FUNCTION_BLOCK Example17_cam //4x3 flyways 2 xbot sample cam set as cam 128 (position interval = 1 mm) - cam mode, cam mode advanced
VAR_INPUT
	Execute : BOOL;
END_VAR
VAR_OUTPUT
	Done : BOOL;
END_VAR
VAR_IN_OUT
	PM_Controller : PMControllerType;	// the planar motor controller to use
END_VAR
VAR
	xbotID_array78 : ARRAY[0..77] OF USINT;
	PosX_array78 : ARRAY[0..77] OF REAL;
	PosY_array78 : ARRAY[0..77] OF REAL;
	PMC_AutoDrivingMotion1 : PMC_AutoDrivingMotion;
	slave_axis_array7 : ARRAY[0..6] OF USINT;
	cam_ID_array7 : ARRAY[0..6] OF USINT;
	master_xbot_ID_array7 : ARRAY[0..6] OF USINT;
	master_axis_array7 : ARRAY[0..6] OF USINT;
	PMC_CamModeCtrl1 : PMC_CamModeCtrl;
	PMC_XYMotion1 : PMC_XYMotion;
	PMC_XYMotion2 : PMC_XYMotion;
	PMC_CamModeCtrl2 : PMC_CamModeCtrl;
	PMC_AutoDrivingMotion2 : PMC_AutoDrivingMotion;
	SlaveAID_array4 : ARRAY[0..3] OF USINT;
	camID_array4 : ARRAY[0..3] OF USINT;
	MasterXID_array4 : ARRAY[0..3] OF USINT;
	MasterAID_array4 : ARRAY[0..3] OF USINT;
	MasterAOffset_array4 : ARRAY[0..3] OF REAL;
	SlaveAOffset_array4 : ARRAY[0..3] OF REAL;
	MasterAScaling_array4 : ARRAY[0..3] OF REAL;
	SlaveAScaling_array4 : ARRAY[0..3] OF REAL;
	CamMode_array4 : ARRAY[0..3] OF USINT;
	MasterOffsetMode_array4 : ARRAY[0..3] OF USINT;
	PMC_CamModeCtrlAdvanced1 : PMC_CamModeCtrlAdvanced;
	PMC_XYMotion3 : PMC_XYMotion;
	PMC_XYMotion4 : PMC_XYMotion;
	PMC_CamModeCtrlAdvanced2 : PMC_CamModeCtrlAdvanced;
END_VAR

//4x3 flyways 2 xbot sample cam set as cam 128 (position interval = 1 mm) - cam mode, cam mode advanced

//move async move to 60,60 and 60,180
xbotID_array78[0] := 1;xbotID_array78[1] := 2;
PosX_array78[0] := 0.06;PosX_array78[1] := 0.06;
PosY_array78[0] := 0.06;PosY_array78[1] := 0.18;
PMC_AutoDrivingMotion1(Execute := Execute,nXbots := 2,XbotID := xbotID_array78,RoutingType := 0,ZoneID := 0,PosX := PosX_array78,PosY := PosY_array78,PM_Controller := PM_Controller);

//setup cam with xbot 2 y as slave to xbot 1 x
slave_axis_array7[0] := 2;
cam_ID_array7[0] := 128;
master_xbot_ID_array7[0] := 1;
master_axis_array7[0] := 1;
PMC_CamModeCtrl1(Execute := PMC_AutoDrivingMotion1.Done,cmdLB := 2,Level := 1,SlaveXID := 2,nAxis := 1,SlaveAID := slave_axis_array7,camID := cam_ID_array7,MasterXID := master_xbot_ID_array7,MasterAID := master_axis_array7,PM_Controller := PM_Controller);

//move xbot 1 to (400,60)
PMC_XYMotion1(Execute := PMC_CamModeCtrl1.Done,cmdLB := 3,XbotID := 1,Mode := 0,Type_ := 0,PosX := 0.4,PosY := 0.06,EndVel := 0,MaxVel := 0.25,MaxAcc := 10,PM_Controller := PM_Controller);

//move xbot 1 to (60,60)
PMC_XYMotion2(Execute := PMC_XYMotion1.Done,cmdLB := 4,XbotID := 1,Mode := 0,Type_ := 0,PosX := 0.06,PosY := 0.06,EndVel := 0,MaxVel := 0.25,MaxAcc := 10,PM_Controller := PM_Controller);

//disable cam on xbot 2 
PMC_CamModeCtrl2(Execute := PMC_XYMotion2.Done,cmdLB := 5,Level := 0,SlaveXID := 2,nAxis := 1,SlaveAID := slave_axis_array7,camID := cam_ID_array7,MasterXID := master_xbot_ID_array7,MasterAID := master_axis_array7,PM_Controller := PM_Controller);

//move to new start position (60,60) and (480,420)
xbotID_array78[0] := 1;xbotID_array78[1] := 2;
PosX_array78[0] := 0.06;PosX_array78[1] := 0.48;
PosY_array78[0] := 0.06;PosY_array78[1] := 0.42;
PMC_AutoDrivingMotion2(Execute := PMC_CamModeCtrl2.Done,nXbots := 2,RoutingType := 0,ZoneID := 0,XbotID := xbotID_array78,PosX := PosX_array78,PosY := PosY_array78,PM_Controller := PM_Controller);

//setup advanced cam
SlaveAID_array4[0] := 1; SlaveAID_array4[1] := 2;
camID_array4[0] := 128; camID_array4[1] := 128;
MasterXID_array4[0] := 1; MasterXID_array4[1] := 1;
MasterAID_array4[0] := 1;MasterAID_array4[1] := 1;
MasterAOffset_array4[0] := 0; MasterAOffset_array4[1] := 0;
SlaveAOffset_array4[0] := 0; SlaveAOffset_array4[1] := 0;
MasterAScaling_array4[0] := 1; MasterAScaling_array4[1] := 2;
SlaveAScaling_array4[0] := 2; SlaveAScaling_array4[1] := 1;
CamMode_array4[0] := 1; CamMode_array4[1] := 1;
MasterOffsetMode_array4[0] := 1; MasterOffsetMode_array4[1] := 1;
PMC_CamModeCtrlAdvanced1(Execute := PMC_AutoDrivingMotion2.Done,cmdLB := 6,Level := 1,SlaveXID := 2,nAxis := 2,SlaveAID := SlaveAID_array4,camID := camID_array4,
						MasterXID := MasterXID_array4,MasterAID := MasterAID_array4,MasterAOffset := MasterAOffset_array4,SlaveAOffset := SlaveAOffset_array4,
						MasterAScaling := MasterAScaling_array4,SlaveAScaling := SlaveAScaling_array4,CamMode := CamMode_array4,MasterOffsetMode := MasterOffsetMode_array4,PM_Controller := PM_Controller);
						
//move xbot 1 to (400,60)
PMC_XYMotion3(Execute := PMC_CamModeCtrlAdvanced1.Done,cmdLB := 7,XbotID := 1,Mode := 0,Type_ := 0,PosX := 0.9,PosY := 0.06,EndVel := 0,MaxVel := 0.25,MaxAcc := 10,PM_Controller := PM_Controller);

//move xbot 1 to (60,60)
PMC_XYMotion4(Execute := PMC_XYMotion3.Done,cmdLB := 8,XbotID := 1,Mode := 0,Type_ := 0,PosX := 0.06,PosY := 0.06,EndVel := 0,MaxVel := 0.25,MaxAcc := 10,PM_Controller := PM_Controller);

//disable advanced cam
PMC_CamModeCtrlAdvanced2(Execute := PMC_XYMotion4.Done,cmdLB := 9,Level := 0,SlaveXID := 2,nAxis := 2,SlaveAID := SlaveAID_array4,camID := camID_array4,
						MasterXID := MasterXID_array4,MasterAID := MasterAID_array4,MasterAOffset := MasterAOffset_array4,SlaveAOffset := SlaveAOffset_array4,
						MasterAScaling := MasterAScaling_array4,SlaveAScaling := SlaveAScaling_array4,CamMode := CamMode_array4,MasterOffsetMode := MasterOffsetMode_array4,PM_Controller := PM_Controller);
						
Done := PMC_CamModeCtrlAdvanced2.Done;

END_FUNCTION_BLOCK
